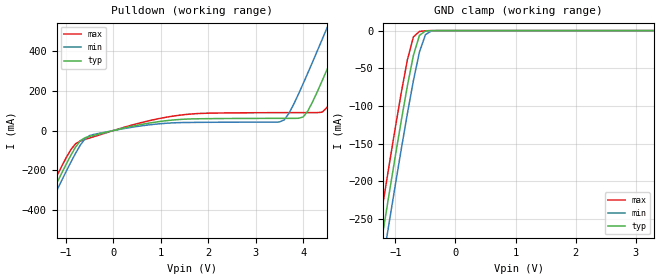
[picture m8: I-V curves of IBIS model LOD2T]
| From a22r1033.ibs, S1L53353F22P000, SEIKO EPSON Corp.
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[Model]   LOD2T
Model_type   Output
Polarity   Non-Inverting
|   typ   min   max
C_comp   5.0pF   4.0pF   6.0pF
|   typ   min   max
[Voltage range]   3.3   3.0   3.6
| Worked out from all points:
|   slope of the pulldown table from 0 to 0.495 V, typ, clamps not added: 18.9 ohm
|   GND clamp passes 1 mA (typ) near -0.51 V on its own axis
[Pulldown]
|   Voltage   I(typ)   I(min)   I(max)
-3.3V     -1.344A    -1.379A    -1.31A
-1.8V     -569.4mA   -606.5mA   -533mA
-1.6V     -467.5mA   -504.9mA   -431mA
-900mV    -125.3mA   -160mA     -97.15mA
-500mV    -29.58mA   -25.14mA   -37.43mA
1.4V      55.64mA    39.77mA    77.15mA
3.6V      61.14mA    53.33mA    89.83mA
4V        67.97mA    235.6mA    89.96mA
4.5V      304.8mA    514.4mA    115.4mA
4.9V      531mA      743.5mA    321.7mA
5.3V      761.4mA    974.8mA    549.5mA
6.6V      1.52A      1.732A     1.307A
[GND_clamp]
|   Voltage   I(typ)   I(min)   I(max)
-3.3V     -1.343A    -1.379A    -1.309A
-1.3V     -314.1mA   -352.4mA   -276.2mA
-1.2V     -264.1mA   -302.5mA   -226.1mA
-1.1V     -214.6mA   -253.1mA   -176.6mA
-1V       -165.9mA   -204.2mA   -128.1mA
-900mV    -118.4mA   -156.3mA   -81.33mA
-800mV    -73.08mA   -109.9mA   -38.6mA
-700mV    -32.75mA   -66.18mA   -8.318mA
-600mV    -6.318mA   -28.41mA   -1.129mA
-500mV    -586.9uA   -5.399mA   -239.5uA
-400mV    -56.77uA   -404.4uA   -18.72uA
3.3V      7.178nA    15.7uA     6.022nA
[Ramp]
|   V_typ   V_min   V_max
dV/dt_r   1.98/0.87n   1.80/1.19n   2.16/0.60n
dV/dt_f   1.98/0.75n   1.80/1.02n   2.16/0.51n
R_load = 5000
